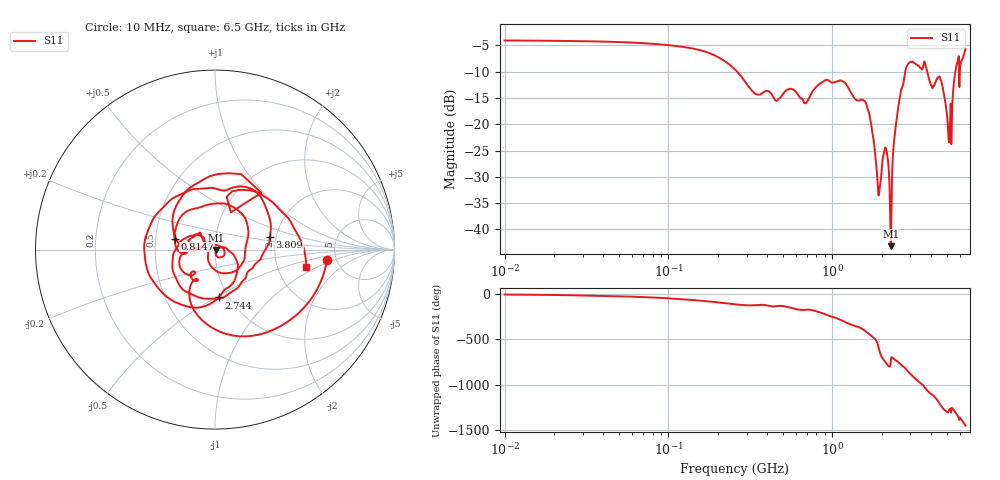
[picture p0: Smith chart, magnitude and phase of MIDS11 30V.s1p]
!Keysight Technologies,E5080B,MY59100498,A.17.05.10
!Date: Wednesday, August 30, 2023 14:18:45
!Correction: S11(C  1-Port  )
!S1P File: Measurement: S11:Log Frequency Sweep
# Hz S  dB  R 50
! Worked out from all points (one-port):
!   1601 points, 10 MHz to 6.5 GHz, reference 50 ohm
!   lowest |S11| = -43.2 dB at 2.278 GHz (marker M1), VSWR 1.01, Z = 50.7 - j0.245 ohm
!   |S11| at or under -10 dB: 263.2 MHz to 2.79 GHz (2.527 GHz wide, 166 % of centre); 3.805 GHz to 5.643 GHz (1.838 GHz wide, 38.9 % of centre); 5.957 GHz to 6.005 GHz (48.35 MHz wide, 0.808 % of centre)
!   S11 on the Smith chart (normalised r, x): 10 MHz: 4.21, -0.79; 814.7 MHz: 0.63, +0.08; 2.744 GHz: 0.90, -0.52; 3.809 GHz: 1.86, +0.28; 6.5 GHz: 2.92, -0.78
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1e7  -4.05 -5.2
2.256172e7  -4.13 -11.2
5.069748e7  -4.36 -24.4
1.139202e8  -5.13 -53.0
2.54951e8  -9.55 -113.4
3.467928e8  -14.31 -121.9
5.728895e8  -13.32 -156.0
6.873597e8  -15.98 -173.3
8.147475e8  -12.62 164.7
1.081653e9  -11.80 88.4
1.292537e9  -13.76 24.7
1.641229e9  -16.86 -66.9
1.92971e9  -33.40 111.0
2.135226e9  -24.68 -42.0
2.278101e9  -43.18 -20.4
2.440395e9  -20.40 -11.3
2.74438e9  -11.46 -85.3
2.904406e9  -8.49 -135.7
3.098749e9  -8.09 171.8
3.373695e9  -8.89 111.9
3.584899e9  -9.11 76.2
3.809325e9  -10.06 12.7
4.371419e9  -11.26 -88.7
4.645083e9  -12.00 -160.8
5.202588e9  -21.94 166.3
5.618531e9  -10.35 140.0
5.946149e9  -7.78 50.8
6.5e9  -5.70 -10.9
